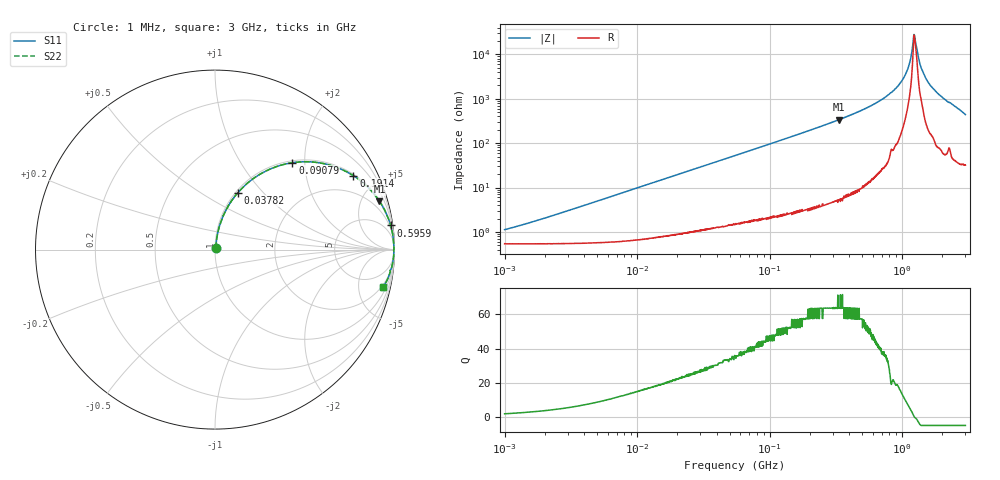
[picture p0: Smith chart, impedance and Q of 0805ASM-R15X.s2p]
!s-Parameter Generated by FASTRON Sdn. Bhd.
!FASTRON P/N : 0805ASM-R15X
!Keysight Technologies: E4991B_MY54100416_A.01.15
!Date: Fri Jun 19 14:50:35 2026
!Version  :Rev00  Fri Jun 19 14:50:35 2026
!Data & Calibration Information:
!Freq  S11  S21  S12  S22
!PortZ  Port1:50+j0  Port2:50+j0
!When reading reference impedance value at option line is always used.
! Remarks : This data is being provided solely for informational purposes.
# Hz S dB R 50
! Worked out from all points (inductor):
!   1601 points, 1 MHz to 3 GHz, reference 50 ohm
!   read as one part in series: L = 157 nH near 1.649 MHz
!   highest Q = 63.8 at 333.5 MHz (marker M1), where L = 162 nH
!   self-resonance near 1.231 GHz
!   S11 on the Smith chart (normalised r, x): 1 MHz: 1.01, +0.02; 37.82 MHz: 1.02, +0.73; 90.79 MHz: 1.04, +1.74; 191.4 MHz: 1.06, +3.71; 595.9 MHz: 1, +14; 3 GHz: 1.64, -8.76
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1000000  -39.00 60.7  -0.05 -0.6  -0.05 -0.6  -39.00 60.7
3804036  -28.50 79.4  -0.05 -2.1  -0.05 -2.1  -28.50 79.4
1.447069e7  -17.10 78.9  -0.15 -8.0  -0.15 -8.0  -17.10 78.9
3.782194e7  -9.39 68.3  -0.64 -19.8  -0.64 -19.8  -9.39 68.3
5.504702e7  -6.71 60.9  -1.17 -27.5  -1.17 -27.5  -6.71 60.9
9.079332e7  -3.76 48.3  -2.54 -40.4  -2.54 -40.4  -3.76 48.3
1.913643e8  -1.17 28.1  -6.53 -60.9  -6.53 -60.9  -1.17 28.1
2.083556e8  -1.00 26.1  -7.14 -63.0  -7.14 -63.0  -1.00 26.1
3.334925e8  -0.40 16.4  -11.00 -72.7  -11.00 -72.7  -0.40 16.4
5.959055e8  -0.11 7.8  -17.30 -80.9  -17.30 -80.9  -0.11 7.8
7.925923e8  -0.05 4.5  -22.00 -83.5  -22.00 -83.5  -0.05 4.5
9.349007e8  -0.04 2.9  -26.00 -83.9  -26.00 -83.9  -0.04 2.9
1.048936e9  -0.03 1.7  -30.50 -82.7  -30.50 -82.7  -0.03 1.7
1.11944e9  -0.03 1.1  -34.70 -80.0  -34.70 -80.0  -0.03 1.1
1.200675e9  -0.03 0.3  -44.10 -62.4  -44.10 -62.4  -0.03 0.3
1.243477e9  -0.03 -0.1  -47.90 13.0  -47.90 13.0  -0.03 -0.1
1.268618e9  -0.04 -0.2  -44.80 40.0  -44.80 40.0  -0.04 -0.2
1.347129e9  -0.03 -0.8  -36.90 75.4  -36.90 75.4  -0.03 -0.8
1.402151e9  -0.04 -1.2  -33.50 78.4  -33.50 78.4  -0.04 -1.2
1.596974e9  -0.04 -2.6  -26.90 82.7  -26.90 82.7  -0.04 -2.6
2.092429e9  -0.09 -5.8  -19.90 81.0  -19.90 81.0  -0.09 -5.8
3e9  -0.35 -12.6  -13.20 73.2  -13.20 73.2  -0.35 -12.6
